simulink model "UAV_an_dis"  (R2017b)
settings: Solver=VariableStepAuto  StartTime=0.0  StopTime=10.0  RelTol=1e-3
libraries: simulink x1

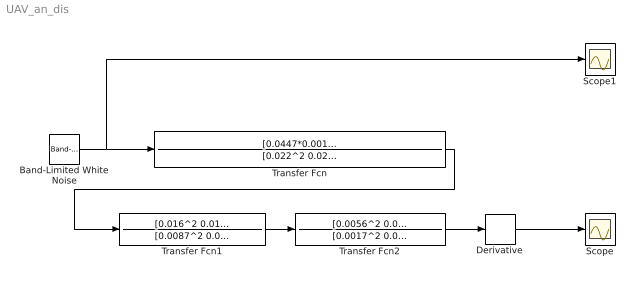
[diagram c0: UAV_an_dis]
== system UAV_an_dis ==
  Band-Limited White Noise : simulink/Sources/Band-Limited White Noise  Cov=[1]  Ts=0.001  seed=[23341]
  Derivative : Derivative
  Scope : Scope
  Scope1 : Scope
  Transfer Fcn : TransferFcn  Numerator=[0.0447*0.0014*0.00031 0.0447*0.00171 0.0447*1]  Denominator=[0.022^2 0.024 1]
  Transfer Fcn1 : TransferFcn  Numerator=[0.016^2 0.013 1]  Denominator=[0.0087^2 0.011 1]
  Transfer Fcn2 : TransferFcn  Numerator=[0.0056^2 0.0074 1]  Denominator=[0.0017^2 0.0021 1]
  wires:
  Band-Limited White Noise/1 -> Scope1/1, Transfer Fcn/1
  Transfer Fcn/1 -> Transfer Fcn1/1
  Transfer Fcn1/1 -> Transfer Fcn2/1
  Transfer Fcn2/1 -> Derivative/1
  Derivative/1 -> Scope/1
